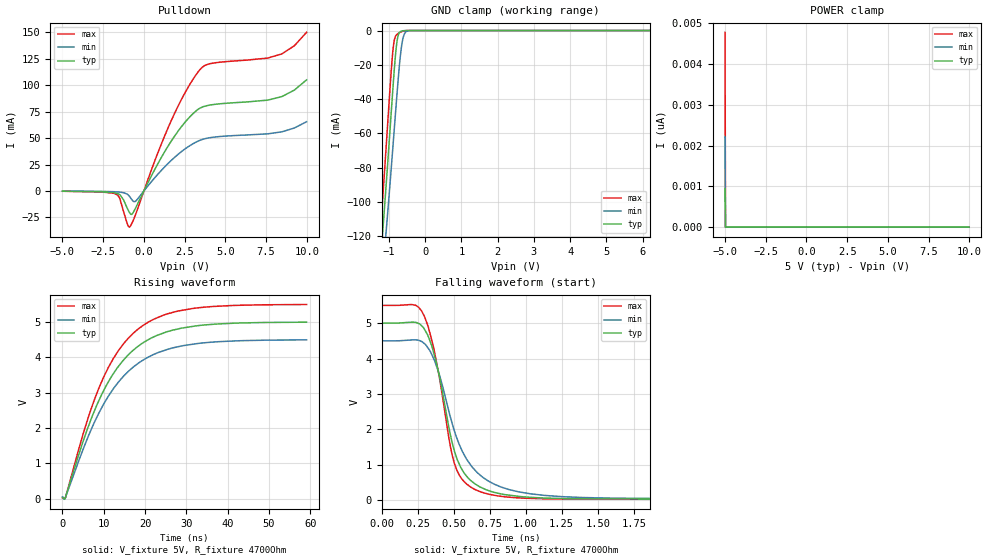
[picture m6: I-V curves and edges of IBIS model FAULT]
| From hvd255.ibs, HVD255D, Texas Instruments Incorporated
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[Model]   FAULT
Model_type   Open_drain
Polarity   Non-Inverting
Vmeas = 2.5
Vref = 2.5
Cref = 15pF
Rref = 4700
|   typ   min   max
|   (nom PVT)   (fast PVT)   (slow PVT)
C_comp   9.3677e-13   9.1552e-13   9.6288e-13
|C_comp (ON state)   9.3745e-13   9.9011e-13   9.4988e-13
|   (nom PVT)   (fast PVT)   (slow PVT)
|C_comp (OFF state)   9.3677e-13   9.1552e-13   9.6288e-13
[Voltage Range]   5   4.5   5.5
[Temperature Range]   27   125   -40
[Pullup Reference]   5   4.5   5.5
[Pulldown Reference]   -0   -0   -0
[Power Clamp Reference]   5   4.5   5.5
[GND Clamp Reference]   -0   -0   -0
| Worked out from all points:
|   slope of the pulldown table from 0 to 0.75 V, typ, clamps not added: 33 ohm
|   GND clamp passes 1 mA (typ) near -0.70 V on its own axis
|   falling waveform, V_fixture 5V, R_fixture 4700Ohm: 20-80 % time 166ps typ, 233ps min, 145ps max; typ from 5 V to 0.033 V
|   rising waveform, V_fixture 5V, R_fixture 4700Ohm: 20-80 % time 12ns typ, 12.5ns min, 11.6ns max; typ from 0.033 V to 5 V
[Pulldown]
|   Voltage   I(typ)   I(min)   I(max)
-5V       -257.5uA   -152.4uA   -297.5uA
-1.775V   -1.824mA   -783.3uA   -2.591mA
-1.505V   -3.213mA   -1.081mA   -6.333mA
-890mV    -20.39mA   -5.07mA    -34.24mA
-740mV    -22.06mA   -8.255mA   -30.61mA
-515mV    -16.24mA   -9.817mA   -22.44mA
1.69V     47.41mA    29.05mA    66.92mA
2.545V    65.37mA    39.98mA    93.48mA
3.43V     78.18mA    47.82mA    114.5mA
4.21V     81.6mA     50.71mA    120.8mA
8.44V     89.11mA    55.84mA    129.5mA
9.985V    105mA      65.43mA    150mA
[GND Clamp]
|   Voltage   I(typ)   I(min)   I(max)
-5V       -891.5mA   -822.5mA   -981.6mA
-1.25V    -140.2mA   -160.9mA   -123.1mA
-1.145V   -111mA     -135.3mA   -90.8mA
-1.04V    -80.28mA   -108.7mA   -57.22mA
-935mV    -48.36mA   -80.92mA   -24.03mA
-875mV    -30.27mA   -64.56mA   -9.427mA
-830mV    -17.84mA   -52.18mA   -4.135mA
-770mV    -5.861mA   -35.9mA    -2.159mA
-650mV    -335.7uA   -9.325mA   -677.9uA
-575mV    -66.54uA   -2.183mA   -194.6uA
-410mV    -670.6nA   -26.16uA   -1.662uA
9.985V    0A         0A         0A
[POWER Clamp]
|   Voltage   I(typ)   I(min)   I(max)
-5V       944.2pA    2.21nA     4.774nA
-4.97V    0A         0A         0A
-4.955V   0A         0A         0A
9.985V    0A         0A         0A
[Ramp]
R_load = 4700
|   typ   min   max
dV/dt_r   2.97832/1.20452e-08   2.66887/1.24535e-08   3.28251/1.16407e-08
dV/dt_f   2.98013/1.66469e-10   2.67098/2.32501e-10   3.28404/1.44621e-10
[Falling Waveform]
V_fixture = 5V
V_fixture_min = 4.5V
V_fixture_max = 5.5V
R_fixture = 4700Ohm
C_fixture = 0F
|   Time   V(typ)   V(min)   V(max)
0s        5V         4.5V       5.5V
236.7ps   5.022V     4.527V     5.503V
297.4ps   4.829V     4.421V     5.192V
383.5ps   3.833V     3.759V     3.846V
491.8ps   1.597V     2.143V     1.245V
572.5ps   772.4mV    1.291V     528.3mV
663.5ps   424.5mV    783mV      277.5mV
782.5ps   222.4mV    453.1mV    141.2mV
1.132ns   62.87mV    137.2mV    40.96mV
59.1ns    33.11mV    48.37mV    26.59mV
[Rising Waveform]
V_fixture = 5V
V_fixture_min = 4.5V
V_fixture_max = 5.5V
R_fixture = 4700Ohm
C_fixture = 0F
|   Time   V(typ)   V(min)   V(max)
0s        33.11mV    48.37mV    26.59mV
426.6ps   -6.667mV   -19.47mV   -1.038mV
744.9ps   46.5mV     40.71mV    32.35mV
6.341ns   2.067V     1.791V     2.335V
9.941ns   3.053V     2.67V      3.435V
13.54ns   3.744V     3.299V     4.191V
18.34ns   4.317V     3.833V     4.805V
24.34ns   4.685V     4.184V     5.191V
31.54ns   4.877V     4.372V     5.385V
59.1ns    4.997V     4.496V     5.497V
